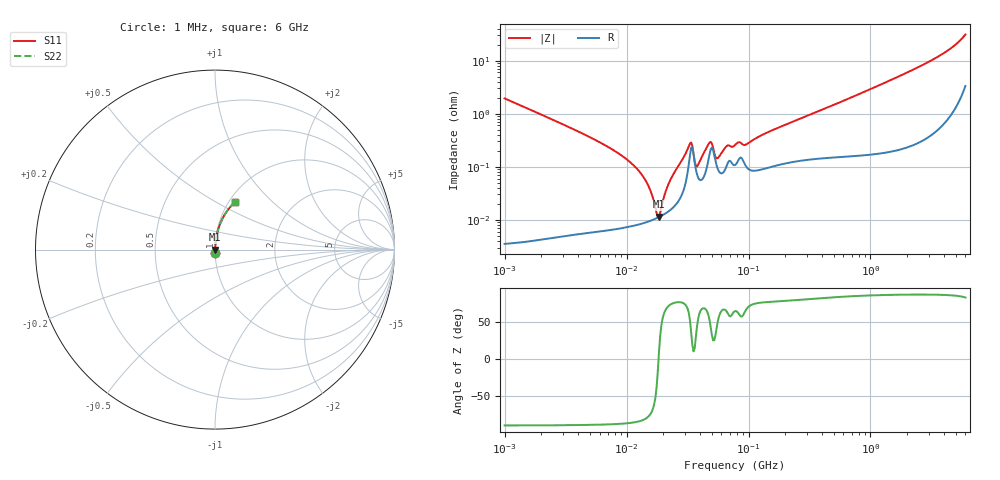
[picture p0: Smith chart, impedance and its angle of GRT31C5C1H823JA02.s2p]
!Murata Part Number: GRT31C5C1H823JA02
!These Parameters are Measured in Series Mode Connection
!Data Generated on Jun 19, 2026
!  o--ll--o
!Port1  Port2
!  o------o
!Operation Temp=25[degC], DC Bias Voltage=0[V]
!Freq. Start=1000[kHz] Stop=6[GHz] 401[Steps]
# Hz S RI R 50
!Freq.(Hz) S11(Real) S11(Imag) S21(Real) S21(Imag) S12(Real) S12(Imag) S22(Real) S22(Imag)
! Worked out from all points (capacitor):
!   401 points, 1 MHz to 6 GHz, reference 50 ohm
!   read as one part in series: C = 81.7 nF near 1.044 MHz
!   lowest |Z| = 11.4 mohm at 18.44 MHz (marker M1)
!   series resonance near 18.29 MHz, so ESL is about 930 pH
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1000000  0.000412 -0.0194  0.9996 0.0194  0.9996 0.0194  0.000412 -0.0194
4293785  7.29e-05 -0.00429  0.9999 0.00429  0.9999 0.00429  7.29e-05 -0.00429
8067822  7.01e-05 -0.00196  0.9999 0.00196  0.9999 0.00196  7.01e-05 -0.00196
1.193364e7  7.98e-05 -0.000958  0.9999 0.000958  0.9999 0.000958  7.98e-05 -0.000958
1.483293e7  9.16e-05 -0.000467  0.9999 0.000467  0.9999 0.000467  9.16e-05 -0.000467
1.618111e7  9.84e-05 -0.000274  0.9999 0.000274  0.9999 0.000274  9.84e-05 -0.000274
1.765184e7  0.000107 -8.02e-05  0.9999 8.02e-05  0.9999 8.02e-05  0.000107 -8.02e-05
1.843659e7  0.000112 1.82e-05  0.9999 -1.82e-05  0.9999 -1.82e-05  0.000112 1.82e-05
2.242276e7  0.000148 0.000491  0.9999 -0.000491  0.9999 -0.000491  0.000148 0.000491
3.316698e7  0.00171 0.00216  0.9983 -0.00216  0.9983 -0.00216  0.00171 0.00216
3.46415e7  0.00231 0.000805  0.9977 -0.000805  0.9977 -0.000805  0.00231 0.000805
3.779011e7  0.000722 0.000702  0.9993 -0.000702  0.9993 -0.000702  0.000722 0.000702
4.800399e7  0.00176 0.00227  0.9982 -0.00227  0.9982 -0.00227  0.00176 0.00227
5.589783e7  0.000913 0.00113  0.9991 -0.00113  0.9991 -0.00113  0.000913 0.00113
6.652088e7  0.00108 0.00223  0.9989 -0.00223  0.9989 -0.00223  0.00108 0.00223
7.745967e7  0.00108 0.00233  0.9989 -0.00233  0.9989 -0.00233  0.00108 0.00233
9.627852e7  0.000992 0.00246  0.999 -0.00246  0.999 -0.00246  0.000992 0.00246
1.424119e8  0.000965 0.00432  0.999 -0.00432  0.999 -0.00432  0.000965 0.00432
3.325952e8  0.00148 0.00981  0.9985 -0.00981  0.9985 -0.00981  0.00148 0.00981
1.428092e9  0.00364 0.0417  0.9964 -0.0417  0.9964 -0.0417  0.00364 0.0417
3.638376e9  0.0195 0.1187  0.9805 -0.1187  0.9805 -0.1187  0.0195 0.1187
6e9  0.1121 0.2664  0.8879 -0.2664  0.8879 -0.2664  0.1121 0.2664
